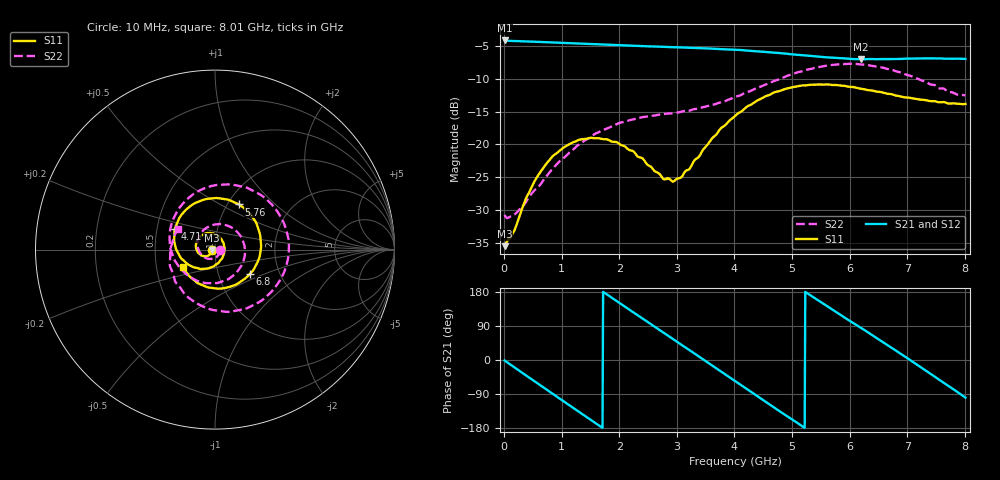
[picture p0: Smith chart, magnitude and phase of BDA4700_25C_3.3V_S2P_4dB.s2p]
!Agilent Technologies,E5071B,MY42404982,A.09.10
!Date: Mon Oct 20 18:04:39 2025
!Data & Calibration Information:
!Freq	S11:SOLT2(ON)	S21:SOLT2(ON)	S12:SOLT2(ON)	S22:SOLT2(ON)
# Hz S RI R 50
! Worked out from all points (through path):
!   801 points, 10 MHz to 8.01 GHz, reference 50 ohm
!   highest |S21| = -4.12 dB at 10 MHz (marker M1); lowest = -7.0 dB at 6.19 GHz (marker M2)
!   group delay of S21, straight-line fit = 283 ps
!   lowest |S11| = -35.5 dB at 10 MHz (marker M3), VSWR 1.03, Z = 48.4 - j0.126 ohm
!   |S11| at or under -10 dB: start of sweep to end of sweep
!   |S22| runs from -31.2 to -7.7 dB; largest |S21 - S12| = 0.0076
!   S11 on the Smith chart (normalised r, x): 10 MHz: 0.97, -0.00; 4.71 GHz: 0.62, +0.15; 5.76 GHz: 1.13, +0.62; 6.8 GHz: 1.41, -0.41; 8.01 GHz: 0.68, -0.14
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1e7  -0.0167 -0.00131  0.622 -0.0134  0.622 -0.0138  0.0289 -0.00251
3.3e8  -0.0245 -0.0235  0.5001 -0.3533  0.5002 -0.3534  0.0198 -0.0275
7.1e8  -0.058 -0.037  0.1551 -0.5838  0.1552 -0.5839  -0.0199 -0.0517
1.02e9  -0.0916 -0.0197  -0.1796 -0.569  -0.1792 -0.569  -0.0694 -0.035
1.35e9  -0.1071 0.0227  -0.4628 -0.3637  -0.4631 -0.3639  -0.0983 0.0317
1.64e9  -0.0915 0.0641  -0.5756 -0.0819  -0.5759 -0.0821  -0.0707 0.1018
1.93e9  -0.0534 0.0899  -0.5324 0.2137  -0.5326 0.2136  0.00783 0.1408
2.32e9  0.00773 0.0805  -0.2661 0.4983  -0.2662 0.4982  0.1254 0.0967
2.68e9  0.0473 0.0377  0.0848 0.5517  0.0843 0.551  0.1666 -0.0253
2.96e9  0.0512 -0.0124  0.3349 0.4386  0.3349 0.4377  0.1255 -0.1201
3.37e9  0.0121 -0.0786  0.5347 0.0994  0.5353 0.0995  -0.0114 -0.1869
3.68e9  -0.0534 -0.1056  0.5 -0.1949  0.5 -0.1967  -0.1279 -0.1586
4.01e9  -0.1388 -0.089  0.3001 -0.4352  0.3007 -0.4343  -0.2202 -0.0667
4.36e9  -0.211 -0.00877  -0.0126 -0.5154  -0.013 -0.5164  -0.2537 0.0809
4.71e9  -0.2245 0.1136  -0.3046 -0.3976  -0.3032 -0.3988  -0.1944 0.2382
5.35e9  -0.042 0.2826  -0.4623 0.1001  -0.4626 0.0976  0.1346 0.3543
5.76e9  0.1331 0.2514  -0.277 0.3641  -0.2764 0.3646  0.3481 0.2108
6.19e9  0.2451 0.1043  0.0354 0.4456  0.0412 0.4464  0.4022 -0.0684
6.68e9  0.2231 -0.0971  0.3584 0.2692  0.3595 0.2685  0.2058 -0.3133
6.8e9  0.1934 -0.1363  0.4067 0.1906  0.408 0.1876  0.1338 -0.3369
7.33e9  0.0106 -0.2171  0.3976 -0.2182  0.3979 -0.2189  -0.1686 -0.2491
8.01e9  -0.18 -0.0957  -0.0732 -0.444  -0.0716 -0.4444  -0.2079 0.1145
